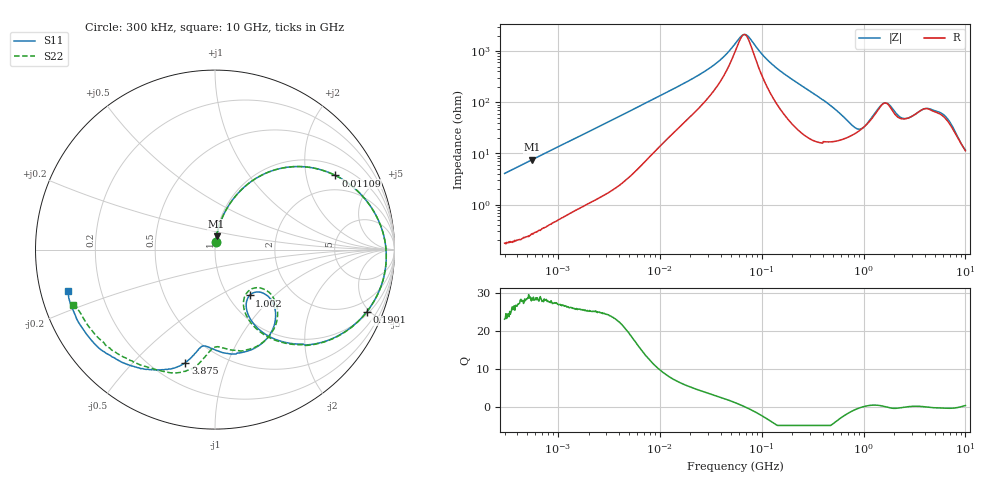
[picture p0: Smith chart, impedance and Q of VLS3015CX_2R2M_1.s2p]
! S-Parameter Data Generated by TDK Corporation
! Copyright(C) 2019 TDK Corporation.
! All Rights Reserved.
! TDK P/N: VLS3015CX-2R2M-1 (Inductor)
! Property: L=2.2uH at 1MHz
! Size(LxWxT): 3x3x1.5mm
! Model Type: s2p (Touchstone File Format Version 1.0)
! Frequency: DC=Yes Start=0.3MHz Stop=10000MHz 802points Log-sweep
! Model Generated on Sep. 23, 2019
! Port Assignments:
!  1 ---@@@--- 2
! Applicable Conditions:
!  Temperature = 25 degC
!  DC Bias Current = 0 A
!  Small Signal Operation
! Terms and conditions regarding TDK Simulation Models
! (1)This simulation model is being provided solely for informational purposes. Please refer to the specifications of the products in terms of detailed characteristics of such products.
! (2)In no event shall TDK Corporation of any of its subsidiaries be liable for any loss or damage arising, directly or indirectly,
!  From any information contained in this simulation model, including, but not limited to loss or damages arising from any inaccuracies, omissions or errors in connection with such information.
! (3)Any and all copyrights on this simulation model are owned by TDK Corporation.
!  Duplication or redistribution of this simulation model without prior written permission from TDK Corporation is prohibited.
! (4)This simulation model is subject to any modification or change without any prior notice.
! (5)Neither TDK Corporation nor any of its subsidiaries shall make any warranty, express or implied,
!  Including but not limited to the correctness, implied warranties of merchantability and fitness for a particular purpose with respect to this simulation models.
! (6)The use of this simulation model shall be deemed to have consented to the terms and conditions hereof.
# Hz S MA R 50
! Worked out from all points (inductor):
!   801 points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, 300 kHz to 10 GHz, reference 50 ohm
!   read as one part in series: L = 2.16 uH near 318.3 kHz
!   highest Q = 28.6 at 561.4 kHz (marker M1), where L = 2.15 uH
!   self-resonance near 67.38 MHz
!   S11 on the Smith chart (normalised r, x): 300 kHz: 1.00, +0.08; 11.09 MHz: 1.36, +2.96; 190.1 MHz: 1.14, -4.79; 1.002 GHz: 1.25, -0.71; 3.875 GHz: 0.33, -0.72; 10 GHz: 0.08, -0.14
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300000  0.04039 85.1  0.9974 -2.3  0.9974 -2.3  0.04026 85.2
561390  0.07527 83.6  0.9945 -4.4  0.9945 -4.4  0.07519 83.6
1713600  0.2204 75.0  0.9668 -12.8  0.9669 -12.8  0.2203 75.0
3777497  0.4385 61.4  0.8797 -26.1  0.8798 -26.1  0.4384 61.4
9671944  0.7543 35.4  0.5857 -48.9  0.5858 -48.9  0.7543 35.4
1.109008e7  0.7879 31.6  0.5324 -51.8  0.5325 -51.8  0.7879 31.6
3.031424e7  0.9237 10.5  0.2039 -63.3  0.2039 -63.3  0.9237 10.4
5.477226e7  0.951 1.3  0.06855 -44.4  0.06858 -44.4  0.9509 1.3
7.160072e7  0.9554 -2.8  0.04686 15.4  0.04687 15.4  0.9554 -2.8
1.063884e8  0.9525 -9.5  0.1226 61.0  0.1226 61.0  0.9525 -9.6
1.900804e8  0.9132 -22.4  0.3008 59.6  0.3009 59.6  0.913 -22.6
3.126428e8  0.8132 -38.1  0.4977 45.3  0.4978 45.3  0.8126 -38.4
4.568044e8  0.6664 -51.5  0.6427 28.8  0.6427 28.8  0.6646 -52.1
6.490631e8  0.4878 -61.9  0.7376 10.1  0.7377 10.1  0.4818 -63.0
1.001841e9  0.3201 -52.9  0.7289 -16.5  0.729 -16.5  0.2987 -53.3
1.307877e9  0.4066 -41.5  0.599 -32.8  0.5992 -32.8  0.385 -38.3
1.767019e9  0.5879 -65.3  0.4515 -27.9  0.4516 -27.9  0.5809 -62.5
2.355454e9  0.5605 -89.6  0.5345 -36.3  0.5344 -36.3  0.5437 -87.1
3.008786e9  0.5459 -97.9  0.4908 -53.8  0.4901 -53.8  0.5717 -93.3
3.874538e9  0.6503 -104.7  0.3668 -65.7  0.3663 -65.7  0.6737 -100.7
6.333834e9  0.8104 -128.7  0.2746 -72.8  0.2746 -72.8  0.7804 -128.5
1e10  0.8535 -164.2  0.239 -92.7  0.2392 -92.8  0.846 -158.8
